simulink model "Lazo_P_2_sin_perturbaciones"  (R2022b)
settings: Solver=ode4  StartTime=0.0  StopTime=0.2  FixedStep=1e-6  RelTol=1e-3
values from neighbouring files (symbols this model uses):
  Ki_P = ((2+3*v_d_2*Kp_P)/(3*v_d_2*tau))    [IP_Lazo_P_2.m]    (also in Sistema_control_no_lineal_LQR.m = ((2+3*v_d_2*Kp_P)/(3*v_d_2*tau_P)); Sistema_control_no_lineal_Modal.m = ((2+3*v_d_2*Kp_P)/(3*v_d_2*tau_P)))
  Kp_P = 1    [IP_Lazo_P_2.m]    (also in Sistema_control_no_lineal_LQR.m = 0.0002; Sistema_control_no_lineal_Modal.m = 0.0002)
  lim_i_d_2_lower = -75.07117    [IP_Lazo_P_2.m]    (also in Sistema_control_no_lineal_LQR.m; Sistema_control_no_lineal_Modal.m)
  lim_i_d_2_upper = 75.07117    [IP_Lazo_P_2.m]    (also in Sistema_control_no_lineal_LQR.m; Sistema_control_no_lineal_Modal.m)
  P_2_1 = -3000    [IP_Lazo_P_2.m]    (also in Sistema_control_no_lineal_LQR.m; Sistema_control_no_lineal_Modal.m)
  P_2_2 = 3000    [IP_Lazo_P_2.m]    (also in Sistema_control_no_lineal_LQR.m; Sistema_control_no_lineal_Modal.m)
  v_d_2 = 100*sqrt(2)    [IP_Lazo_P_2.m]    (also in Sistema_no_lineal_Modal.m; Sistema_no_lineal_LQR.m; Sistema_control_no_lineal_LQR.m; Sistema_control_no_lineal_Modal.m)

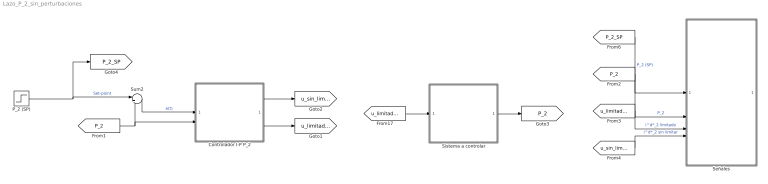
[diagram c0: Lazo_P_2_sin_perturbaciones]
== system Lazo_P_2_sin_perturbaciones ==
  Controlador I-P P_2 : Subsystem
  P_2 (SP) : Step  Time=0.1  Before=P_2_1  After=P_2_2  SampleTime=0
  Señales : Subsystem
  Sistema a controlar : Subsystem
  Sum2 : Sum  Inputs=|+-
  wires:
  P_2 (SP)/1 -> [P_2_SP], Sum2/1  "Set-point"
  Sum2/1 -> Controlador I-P P_2/1(e(t))  "e(t)"
  Controlador I-P P_2/2(i^d*_2 limitado) -> [u_limitado_2]
  Controlador I-P P_2/1(i^d*_2 sin limitar) -> [u_sin_limitar_2]
  [u_limitado_2] -> Sistema a controlar/1(i^d*_2 limitado)
  Sistema a controlar/1(P_2) -> [P_2]
  [P_2_SP] -> Señales/1(P_2 (SP))  "P_2 (SP)"
  [P_2] -> Señales/2(P_2)  "P_2"
  [u_limitado_2] -> Señales/3(i^d*_2 limitado)  "i^d*_2 limitado"
  [u_sin_limitar_2] -> Señales/4(i^d*_2 sin limitar)  "i^d*_2 sin limitar"
  [P_2] -> Controlador I-P P_2/2(P_2), Sum2/2

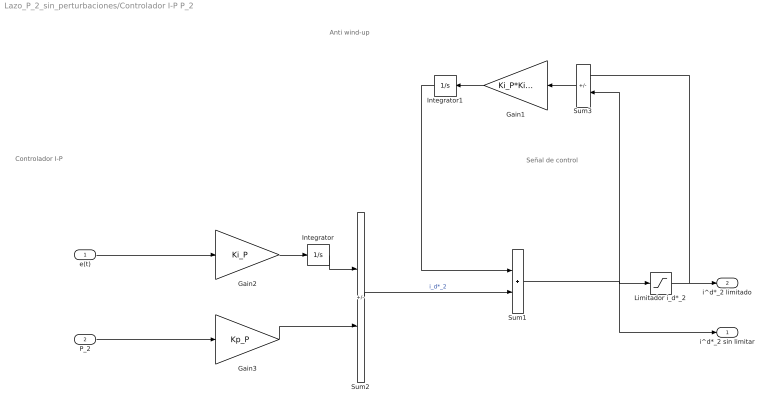
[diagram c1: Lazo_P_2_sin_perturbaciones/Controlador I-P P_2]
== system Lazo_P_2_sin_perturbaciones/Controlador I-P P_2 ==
  note: Señal de control
  note: Controlador I-P
  note: Anti wind-up
  e(t) : Inport
  P_2 : Inport  Port=2
  Gain1 : Gain  Gain=Ki_P*Ki_P
  Gain2 : Gain  Gain=Ki_P
  Gain3 : Gain  Gain=Kp_P
  Integrator : Integrator
  Integrator1 : Integrator
  Limitador i_d*_2 : Saturate  UpperLimit=lim_i_d_2_upper  LowerLimit=lim_i_d_2_lower
  Sum1 : Sum
  Sum2 : Sum  Inputs=+-
  Sum3 : Sum  Inputs=+-
  i^d*_2 sin limitar : Outport
  i^d*_2 limitado : Outport  Port=2
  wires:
  Limitador i_d*_2/1 -> i^d*_2 limitado/1, Sum3/1
  Sum1/1 -> i^d*_2 sin limitar/1, Limitador i_d*_2/1, Sum3/2
  Sum2/1 -> Sum1/2  "i_d*_2"
  Gain2/1 -> Integrator/1
  Integrator/1 -> Sum2/1
  e(t)/1 -> Gain2/1
  Sum3/1 -> Gain1/1
  Gain1/1 -> Integrator1/1
  Integrator1/1 -> Sum1/1
  P_2/1 -> Gain3/1
  Gain3/1 -> Sum2/2

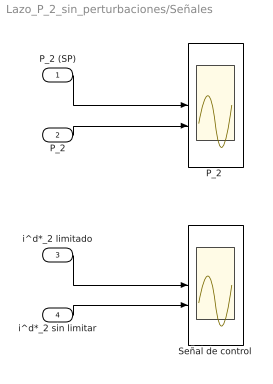
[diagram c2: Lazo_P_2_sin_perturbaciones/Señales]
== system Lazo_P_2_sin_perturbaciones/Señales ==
  P_2 (SP) : Inport
  P_2 : Inport  Port=2
  i^d*_2 limitado : Inport  Port=3
  i^d*_2 sin limitar : Inport  Port=4
  "P_2 " : Scope  NumInputPorts=2
  Señal de control : Scope  NumInputPorts=2
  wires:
  P_2 (SP)/1 -> "P_2 "/1
  i^d*_2 sin limitar/1 -> Señal de control/2
  i^d*_2 limitado/1 -> Señal de control/1
  P_2/1 -> "P_2 "/2

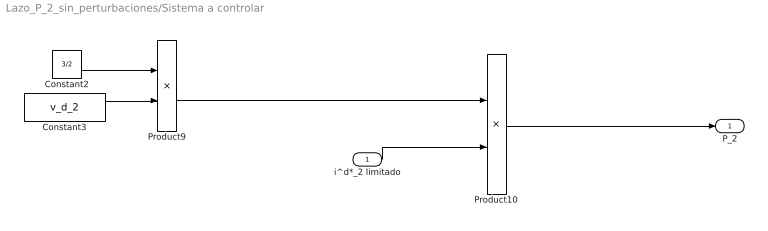
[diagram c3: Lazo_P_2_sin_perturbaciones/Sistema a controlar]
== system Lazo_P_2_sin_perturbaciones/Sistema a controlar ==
  i^d*_2 limitado : Inport
  Constant2 : Constant  Value=3/2
  Constant3 : Constant  Value=v_d_2
  Product10 : Product
  Product9 : Product
  P_2 : Outport
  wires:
  Product9/1 -> Product10/1
  i^d*_2 limitado/1 -> Product10/2
  Constant3/1 -> Product9/2
  Constant2/1 -> Product9/1
  Product10/1 -> P_2/1
